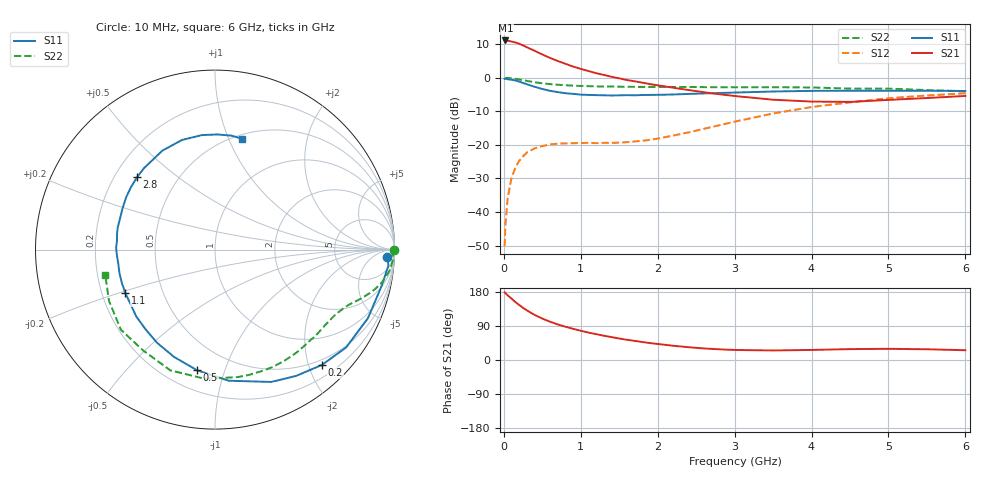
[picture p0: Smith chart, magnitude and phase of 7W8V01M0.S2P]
! Infineon Technologies  Discrete & RF Semiconductors
! BFS17W
! Si NPN RF Bipolar Junction Transistor in SOT323
! VCE = 8 V  IC = 1 mA
! Common Emitter S-Parameters:  August  1999
# GHz  S  MA  R  50
!  f  S11  S21  S12  S22
! GHz  MAG  ANG  MAG  ANG  MAG  ANG  MAG  ANG
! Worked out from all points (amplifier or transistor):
!   36 points, 10 MHz to 6 GHz, reference 50 ohm
!   highest |S21| = 11.1 dB at 20 MHz (marker M1)
!   |S21| within 3 dB of that: start of sweep to 392.5 MHz
!   unconditionally stable (mu >= 1): 1.075 GHz to 3.285 GHz; 4.011 GHz to end of sweep
!   at 250 MHz: K = 0.25, MSG = 16.5 dB, |S12| = -23.4 dB
!   at 1.4 GHz: K = 1.23, MAG = 6.9 dB, |S12| = -19.4 dB
!   at 6 GHz: K = 1.08, MAG = -2.2 dB, |S12| = -4.6 dB
!   S11 on the Smith chart (normalised r, x): 10 MHz: 25, -25; 200 MHz: 0.40, -2.23; 500 MHz: 0.32, -0.81; 1.1 GHz: 0.30, -0.21; 2.8 GHz: 0.29, +0.36; 6 GHz: 0.54, +1.12
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0.01  0.9603 -2.3  3.586 178.8  0.0031 81.8  0.9999 -0.1
0.02  0.9705 -5.2  3.595 176.4  0.0063 89.8  0.9898 -1.3
0.05  0.9503 -12.3  3.57 170.7  0.0162 85.5  0.9935 -3.2
0.1  0.9338 -24.2  3.46 162.0  0.0322 76.4  0.9825 -6.4
0.15  0.9116 -36.7  3.36 153.0  0.0459 69.5  0.9635 -9.2
0.2  0.8764 -47.1  3.207 145.0  0.058 64.2  0.9428 -11.6
0.25  0.8365 -57.3  3.033 137.6  0.0677 58.6  0.9192 -13.8
0.3  0.801 -67.0  2.847 130.9  0.077 54.3  0.8985 -15.5
0.4  0.7344 -84.1  2.522 118.9  0.0889 47.0  0.8584 -18.5
0.5  0.6799 -98.4  2.223 109.4  0.0961 42.2  0.8274 -20.7
0.6  0.64 -110.9  1.975 101.0  0.1014 38.6  0.8047 -22.6
0.7  0.6111 -122.0  1.78 94.0  0.1045 36.6  0.7873 -24.5
0.9  0.5755 -139.7  1.47 82.3  0.106 34.5  0.7627 -28.3
1.1  0.5551 -154.2  1.26 72.3  0.1072 35.6  0.7497 -32.3
1.6  0.5512 178.8  0.925 53.3  0.1099 45.3  0.7332 -43.4
2.2  0.5635 156.2  0.711 37.6  0.1375 62.0  0.7298 -58.5
2.8  0.5924 137.1  0.569 28.2  0.1961 70.0  0.7235 -74.8
3.5  0.6243 118.1  0.471 25.1  0.2934 68.7  0.7222 -94.4
4  0.6378 106.8  0.442 26.6  0.3665 63.3  0.7173 -110.3
4.5  0.6423 96.6  0.437 28.7  0.4297 56.4  0.6899 -125.5
5.5  0.6416 81.7  0.499 28.3  0.5446 42.4  0.6561 -154.2
6  0.6355 76.2  0.536 25.8  0.5883 35.7  0.6277 -166.9
